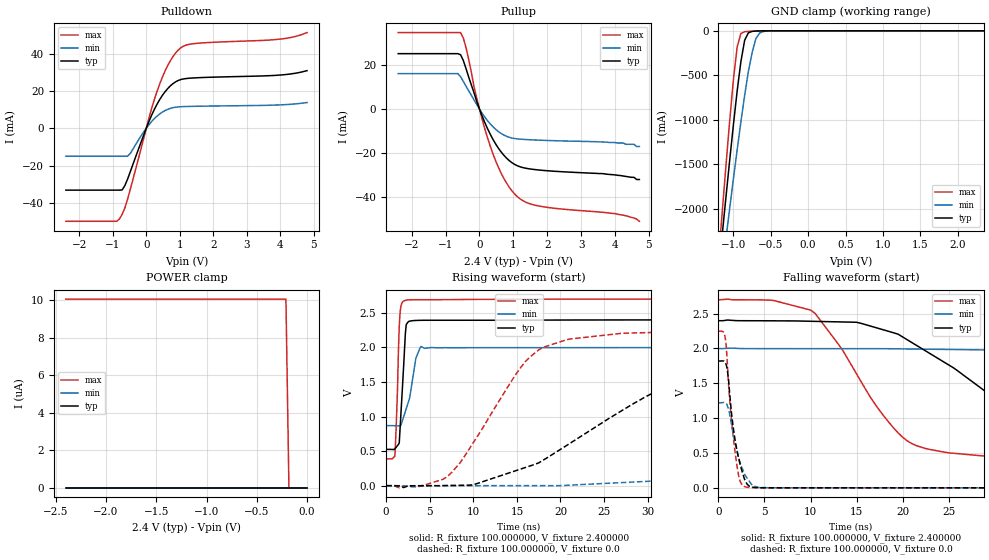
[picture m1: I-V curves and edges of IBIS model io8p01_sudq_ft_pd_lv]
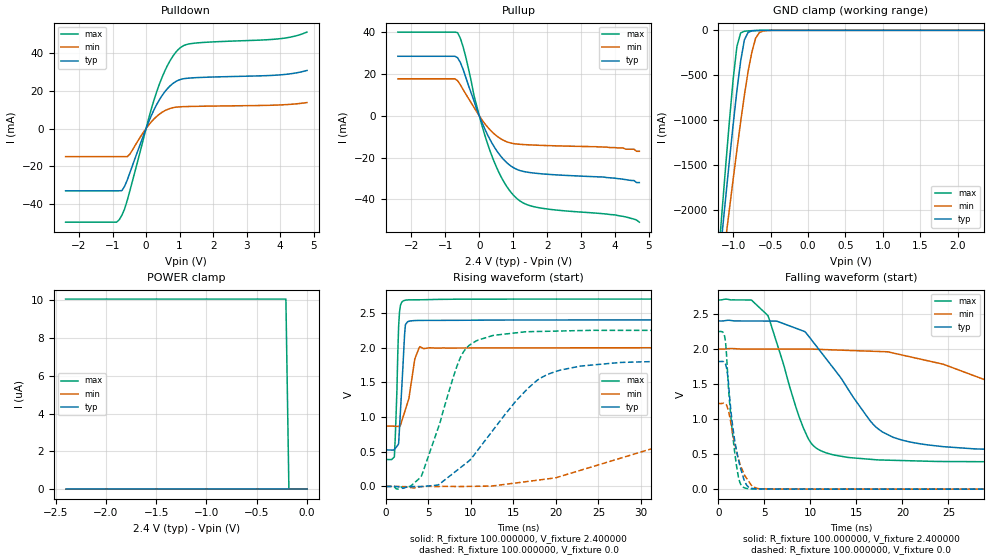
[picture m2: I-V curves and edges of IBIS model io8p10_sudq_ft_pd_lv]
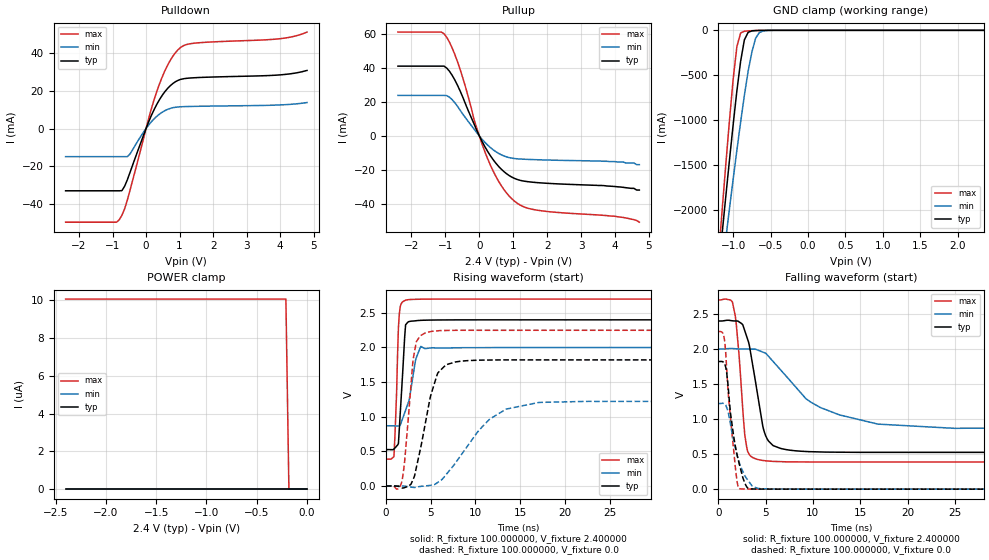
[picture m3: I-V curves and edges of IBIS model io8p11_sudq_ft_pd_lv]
|   stm32f0_444_lqfp32 IBIS Model
[IBIS ver]   4.2
[File name]  stm32f0_444_lqfp32.ibs
[File Rev]   1.0
[Date]   15-5-2013
[Source] Data Created at STMicroelectronics
[Notes]   File originated from ELDO simulations.
[Disclaimer]  This information is for modeling purpose only and is
   not guaranted. The information is subject to change without
   notice.
[Copyright] Copyright 2015 STMicroelectronics Inc.
[Component] stm32f0_444_lqfp32
[Manufacturer] STMicroelectronics
[Package]
| variable   typ   min   max
R_pkg   0.0   NA   NA
L_pkg   0.0H   NA   NA
C_pkg   0.0F   NA   NA
[Pin] signal_name  model_name   R_pin   L_pin   C_pin
1   VDD   POWER   0.03449   2.11E-09   6E-14
2   PF0   io8p_sudq_ft   0.029020556   1.54333E-09   3.22222E-14
3   PF1   io8p_sudq_ft   0.025738889   1.20333E-09   1.55556E-14
4   NRST   ioreset_tc_v33   0.024645   1.09E-09   1E-14
5   VDDA   POWER   0.024645   1.09E-09   1E-14
6   PA0   io8p_sudq_ft   0.025738889   1.20333E-09   1.55556E-14
7   PA1   io8p_sudq_ft   0.029020556   1.54333E-09   3.22222E-14
8   PA2   io8p_sudq_ft   0.03449   2.11E-09   6E-14
9   PA3   io8p_sudq_ft   0.03449   2.11E-09   6E-14
10   PA4   io8p_sudq_ft   0.029020556   1.54333E-09   3.22222E-14
11   PA5   io8p_sudq_ft   0.025738889   1.20333E-09   1.55556E-14
12   PA6   io8p_sudq_ft   0.024645   1.09E-09   1E-14
13   PA7   io8p_sudq_ft   0.024645   1.09E-09   1E-14
14   PB0   io8p_sudq_ft   0.025738889   1.20333E-09   1.55556E-14
15   PB1   io8p_sudq_ft   0.029020556   1.54333E-09   3.22222E-14
16   VSS   GND   0.03449   2.11E-09   6E-14
17   VDD   POWER   0.03449   2.11E-09   6E-14
18   PA8   io8p_sudq_ft   0.029020556   1.54333E-09   3.22222E-14
19   PA9   io8p_sudq_ft   0.025738889   1.20333E-09   1.55556E-14
20   PA10   io8p_sudq_ft   0.024645   1.09E-09   1E-14
21   PA11   io8p_sudq_ft   0.024645   1.09E-09   1E-14
22   PA12   io8p_sudq_ft   0.025738889   1.20333E-09   1.55556E-14
23   PA13   io8p_sudq_ft   0.029020556   1.54333E-09   3.22222E-14
24   PA14   io8p_sudq_ft   0.03449   2.11E-09   6E-14
25   PA15   io8p_sudq_ft   0.03449   2.11E-09   6E-14
26   PB3   io8p_sudq_ft   0.029020556   1.54333E-09   3.22222E-14
27   PB4   io8p_sudq_ft   0.025738889   1.20333E-09   1.55556E-14
28   PB5   io8p_sudq_ft   0.024645   1.09E-09   1E-14
29   PB6   io8p_sudq_i2cin_lv_ft   0.024645   1.09E-09   1E-14
30   PB7   io8p_sudq_i2cin_lv_ft   0.025738889   1.20333E-09   1.55556E-14
31   BOOT0   vpp_test_hv   0.029020556   1.54333E-09   3.22222E-14
32   VSS   GND   0.03449   2.11E-09   6E-14
[Model Selector] io8p_sudq_ft
io8p01_sudq_ft_pd_lv  "SPEED01 2P0V, PD=40kOhm"
io8p01_sudq_ft_pu_lv  "SPEED01 2P0V, PU=40kOhm"
io8p01_sudq_ft_lv  "SPEED01 2P0V"
io8p10_sudq_ft_pd_lv  "SPEED10 2P0V, PD=40kOhm"
io8p10_sudq_ft_pu_lv  "SPEED10 2P0V, PU=40kOhm"
io8p10_sudq_ft_lv  "SPEED10 2P0V"
io8p11_sudq_ft_pd_lv  "SPEED11 2P0V, PD=40kOhm"
io8p11_sudq_ft_pu_lv  "SPEED11 2P0V, PU=40kOhm"
io8p11_sudq_ft_lv  "SPEED11 2P0V"
io8p01_sudq_ft_pd  "SPEED01, PD=40kOhm"
io8p01_sudq_ft_pu  "SPEED01, PU=40kOhm"
io8p01_sudq_ft  "SPEED01"
io8p10_sudq_ft_pd  "SPEED10, PD=40kOhm"
io8p10_sudq_ft_pu  "SPEED10, PU=40kOhm"
io8p10_sudq_ft  "SPEED10"
io8p11_sudq_ft_pd  "SPEED11, PD=40kOhm"
io8p11_sudq_ft_pu  "SPEED11, PU=40kOhm"
io8p11_sudq_ft  "SPEED11"
[Model Selector] io8p_sudq_i2cin_lv_ft
io8p01_sudq_i2cin_lv_ft_pd_lv  "SPEED01 2P0V, PD=40kOhm"
io8p01_sudq_i2cin_lv_ft_pu_lv  "SPEED01 2P0V, PU=40kOhm"
io8p01_sudq_i2cin_lv_ft_lv  "SPEED01 2P0V"
io8p10_sudq_i2cin_lv_ft_pd_lv  "SPEED10 2P0V, PD=40kOhm"
io8p10_sudq_i2cin_lv_ft_pu_lv  "SPEED10 2P0V, PU=40kOhm"
io8p10_sudq_i2cin_lv_ft_lv  "SPEED10 2P0V"
io8p11_sudq_i2cin_lv_ft_pd_lv  "SPEED11 2P0V, PD=40kOhm"
io8p11_sudq_i2cin_lv_ft_pu_lv  "SPEED11 2P0V, PU=40kOhm"
io8p11_sudq_i2cin_lv_ft_lv  "SPEED11 2P0V"
io8p01_sudq_i2cin_lv_ft_pd  "SPEED01, PD=40kOhm"
io8p01_sudq_i2cin_lv_ft_pu  "SPEED01, PU=40kOhm"
io8p01_sudq_i2cin_lv_ft  "SPEED01"
io8p10_sudq_i2cin_lv_ft_pd  "SPEED10, PD=40kOhm"
io8p10_sudq_i2cin_lv_ft_pu  "SPEED10, PU=40kOhm"
io8p10_sudq_i2cin_lv_ft  "SPEED10"
io8p11_sudq_i2cin_lv_ft_pd  "SPEED11, PD=40kOhm"
io8p11_sudq_i2cin_lv_ft_pu  "SPEED11, PU=40kOhm"
io8p11_sudq_i2cin_lv_ft  "SPEED11"
[Model Selector] ioreset_tc_v33
ioreset_tc_v33_pu_lv  "IORESET 2V + PU=40kOhm"
ioreset_tc_v33_nopu_lv  "IORESET 2V"
ioreset_tc_v33_pu  "IORESET + PU=40kOhm"
ioreset_tc_v33_nopu  "IORESET"
[Model Selector] vpp_test_hv
vpp_test_hv_3p3  "Input Buffer"
vpp_test_hv_2p4  "Input Buffer 2P0V"
| Models and submodels in the file (42): io8p01_sudq_ft_pd_lv (I/O), io8p01_sudq_ft_pu_lv (I/O), io8p01_sudq_ft_lv (I/O), io8p10_sudq_ft_pd_lv (I/O), io8p10_sudq_ft_pu_lv (I/O), io8p10_sudq_ft_lv (I/O), io8p11_sudq_ft_pd_lv (I/O), io8p11_sudq_ft_pu_lv (I/O), io8p11_sudq_ft_lv (I/O), io8p01_sudq_ft_pd (I/O), io8p01_sudq_ft_pu (I/O), io8p01_sudq_ft (I/O), io8p10_sudq_ft_pd (I/O), io8p10_sudq_ft_pu (I/O), io8p10_sudq_ft (I/O), io8p11_sudq_ft_pd (I/O), io8p11_sudq_ft_pu (I/O), io8p11_sudq_ft (I/O), io8p01_sudq_i2cin_lv_ft_pd_lv (I/O), io8p01_sudq_i2cin_lv_ft_pu_lv (I/O), io8p01_sudq_i2cin_lv_ft_lv (I/O), io8p10_sudq_i2cin_lv_ft_pd_lv (I/O), io8p10_sudq_i2cin_lv_ft_pu_lv (I/O), io8p10_sudq_i2cin_lv_ft_lv (I/O), io8p11_sudq_i2cin_lv_ft_pd_lv (I/O), io8p11_sudq_i2cin_lv_ft_pu_lv (I/O), io8p11_sudq_i2cin_lv_ft_lv (I/O), io8p01_sudq_i2cin_lv_ft_pd (I/O), io8p01_sudq_i2cin_lv_ft_pu (I/O), io8p01_sudq_i2cin_lv_ft (I/O), io8p10_sudq_i2cin_lv_ft_pd (I/O), io8p10_sudq_i2cin_lv_ft_pu (I/O), io8p10_sudq_i2cin_lv_ft (I/O), io8p11_sudq_i2cin_lv_ft_pd (I/O), io8p11_sudq_i2cin_lv_ft_pu (I/O), io8p11_sudq_i2cin_lv_ft (I/O), ioreset_tc_v33_pu_lv (I/O_open_drain), ioreset_tc_v33_nopu_lv (I/O_open_drain), ioreset_tc_v33_pu (I/O_open_drain), ioreset_tc_v33_nopu (I/O_open_drain), vpp_test_hv_2p4 (Input), vpp_test_hv_3p3 (Input)
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|   Model io8p01_sudq_ft_pd_lv
[Model]  io8p01_sudq_ft_pd_lv
Model_type I/O
Polarity   Non-Inverting
Enable   Active-Low
Vinl =   0.720000V
Vinh =   1.680000V
Vmeas =  1.200000V
Cref =   50.000000pF
Rref =   100.000000M
Vref =   0.0V
C_comp   1.970100pF   1.887900pF   2.069400pF
[Temperature Range]   25.000000   0.125000k   -40.000000
[Pullup Reference]   2.400000V   2.000000V   2.700000V
[Pulldown Reference]   0.0V   0.0V   0.0V
[POWER Clamp Reference]   2.400000V   2.000000V   2.700000V
[GND Clamp Reference]   0.0V   0.0V   0.0V
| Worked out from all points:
|   slope of the pulldown table from 0 to 0.36 V, typ, clamps not added: 25.5 ohm
|   slope of the pullup table from 0 to 0.36 V, typ, clamps not added: 28.4 ohm
|   GND clamp passes 1 mA (typ) near -0.64 V on its own axis
|   rising waveform, R_fixture 100.000000, V_fixture 2.400000: 20-80 % time 499ps typ, 1.06ns min, 336ps max; typ from 0.525 V to 2.4 V
|   rising waveform, R_fixture 100.000000, V_fixture 0.0: 20-80 % time 14.6ns typ, 43.7ns min, 6.88ns max; typ from 0 V to 1.82 V
|   falling waveform, R_fixture 100.000000, V_fixture 2.400000: 20-80 % time 12.9ns typ, 32.5ns min, 7.07ns max; typ from 2.4 V to 0.525 V
|   falling waveform, R_fixture 100.000000, V_fixture 0.0: 20-80 % time 1.15ns typ, 1.36ns min, 910ps max; typ from 1.82 V to 0 V
[Pulldown]
|Voltage   I(typ)   I(min)   I(max)
-2.4V     -33.16mA   -14.98mA   -49.86mA
-880mV    -33.16mA   -14.98mA   -49.86mA
-800mV    -33.16mA   -14.98mA   -48.55mA
-640mV    -30.75mA   -14.98mA   -42.76mA
-480mV    -23.43mA   -13.57mA   -32.92mA
80mV      3.651mA    1.905mA    5.506mA
400mV     15.37mA    7.665mA    23.73mA
720mV     22.75mA    10.69mA    36.23mA
1.04V     26.18mA    11.57mA    43.27mA
1.52V     27.09mA    11.81mA    45.55mA
4V        28.55mA    12.55mA    47.81mA
4.8V      30.9mA     13.81mA    51.31mA
[Pullup]
|Voltage   I(typ)   I(min)   I(max)
-2.4V     25.2mA     16.13mA    34.79mA
-640mV    25.2mA     16.13mA    34.79mA
-560mV    24.71mA    14.75mA    34.79mA
-400mV    18.51mA    10.48mA    28.09mA
-160mV    7.338mA    4.152mA    10.02mA
80mV      -3.229mA   -1.94mA    -4.736mA
400mV     -13.82mA   -8.081mA   -20.45mA
800mV     -22.31mA   -12.38mA   -33.66mA
1.2V      -26.24mA   -13.65mA   -40.83mA
1.76V     -27.69mA   -14.12mA   -44.07mA
4V        -29.9mA    -15.2mA    -47.5mA
4.72V     -32mA      -17mA      -51mA
[GND_clamp]
|Voltage   I(typ)   I(min)   I(max)
-2.4V     -9.788A    -9.782A    -9.734A
-1.2V     -2.718A    -3.021A    -2.568A
-1.15V    -2.29A     -2.675A    -2.036A
-1.1V     -1.868A    -2.333A    -1.515A
-1.05V    -1.454A    -1.995A    -1.012A
-950mV    -674.5mA   -1.337A    -180.6mA
-900mV    -345.2mA   -1.023A    -29.74mA
-850mV    -106.4mA   -726mA     -10.14mA
-750mV    -6.411mA   -244mA     -4.042mA
-700mV    -2.572mA   -88.62mA   -2.346mA
-600mV    -429.6uA   -7.75mA    -383.5uA
2.35V     59.77uA    46.33uA    66.89uA
[POWER_clamp]
|Voltage   I(typ)   I(min)   I(max)
-2.4V     0A         0A         10.06uA
-210mV    0A         0A         10.06uA
-180mV    0A         0A         0A
0V        0A         0A         0A
[Ramp]
| variable   typ   min   max
dV/dt_r  1.09218/14.55718n   0.73266/43.64565n   1.34874/6.87247n
dV/dt_f  1.12429/12.86053n   0.67801/32.45722n   1.38701/7.06387n
R_load = 100.000000
[Rising Waveform]
R_fixture= 100.000000
V_fixture= 2.400000
V_fixture_min= 2.000000
V_fixture_max= 2.700000
|time   V(typ)   V(min)   V(max)
0s        524.8mV    868.7mV    387.2mV
1.001ns   533mV      867mV      427.7mV
1.301ns   579.7mV    865.4mV    1.395V
1.502ns   618.4mV    864.7mV    2.307V
1.602ns   837.8mV    864.4mV    2.512V
2.102ns   1.961V     1.034V     2.677V
2.302ns   2.331V     1.113V     2.684V
3.403ns   2.39V      1.843V     2.691V
4.004ns   2.392V     2.014V     2.691V
49.85ns   2.399V     1.999V     2.699V
[Rising Waveform]
R_fixture= 100.000000
V_fixture= 0.0
V_fixture_min= 0.0
V_fixture_max= 0.0
|time   V(typ)   V(min)   V(max)
0s        1.768nV    15.89nV    1.355nV
7.007ns   1.867mV    822uV      130.1mV
15.02ns   222.8mV    610.6uV    1.635V
17.52ns   330.7mV    351.7uV    1.966V
27.03ns   1.085V     44.44mV    2.204V
34.53ns   1.55V      90.81mV    2.229V
43.04ns   1.723V     239mV      2.246V
84.08ns   1.82V      945.5mV    2.248V
103.1ns   1.82V      1.111V     2.248V
249.2ns   1.82V      1.221V     2.248V
[Falling Waveform]
R_fixture= 100.000000
V_fixture= 2.400000
V_fixture_min= 2.000000
V_fixture_max= 2.700000
|time   V(typ)   V(min)   V(max)
0s        2.399V     1.999V     2.699V
10.01ns   2.391V     1.998V     2.551V
15.02ns   2.376V     1.997V     1.633V
20.02ns   2.165V     1.994V     725.2mV
29.53ns   1.332V     1.979V     449.6mV
35.04ns   877.6mV    1.964V     425.1mV
42.54ns   673.2mV    1.851V     405.8mV
67.07ns   552.7mV    1.286V     389.2mV
85.59ns   536.1mV    1.035V     387.2mV
249.2ns   524.8mV    868.7mV    387.2mV
[Falling Waveform]
R_fixture= 100.000000
V_fixture= 0.0
V_fixture_min= 0.0
V_fixture_max= 0.0
|time   V(typ)   V(min)   V(max)
0s        1.82V      1.221V     2.248V
700.7ps   1.801V     1.221V     2.178V
800.8ps   1.783V     1.214V     2.095V
1.001ns   1.652V     1.164V     1.701V
1.401ns   1.088V     921.6mV    989mV
1.802ns   687.3mV    646.2mV    513.2mV
2.302ns   364.2mV    381.5mV    115.5mV
2.903ns   104.2mV    178.7mV    14.94mV
4.705ns   1.559mV    3.204mV    789.6uV
49.85ns   1.768nV    15.89nV    1.355nV
|   Model io8p10_sudq_ft_pd_lv
[Model]  io8p10_sudq_ft_pd_lv
Model_type I/O
Polarity   Non-Inverting
Enable   Active-Low
Vinl =   0.720000V
Vinh =   1.680000V
Vmeas =  1.200000V
Cref =   50.000000pF
Rref =   100.000000M
Vref =   0.0V
C_comp   1.970100pF   1.887900pF   2.069400pF
[Temperature Range]   25.000000   0.125000k   -40.000000
[Pullup Reference]   2.400000V   2.000000V   2.700000V
[Pulldown Reference]   0.0V   0.0V   0.0V
[POWER Clamp Reference]   2.400000V   2.000000V   2.700000V
[GND Clamp Reference]   0.0V   0.0V   0.0V
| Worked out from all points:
|   slope of the pulldown table from 0 to 0.36 V, typ, clamps not added: 25.5 ohm
|   slope of the pullup table from 0 to 0.36 V, typ, clamps not added: 28.4 ohm
|   GND clamp passes 1 mA (typ) near -0.64 V on its own axis
|   rising waveform, R_fixture 100.000000, V_fixture 2.400000: 20-80 % time 501ps typ, 1.06ns min, 337ps max; typ from 0.525 V to 2.4 V
|   rising waveform, R_fixture 100.000000, V_fixture 0.0: 20-80 % time 7.37ns typ, 21.8ns min, 3.53ns max; typ from 0 V to 1.82 V
|   falling waveform, R_fixture 100.000000, V_fixture 2.400000: 20-80 % time 6.27ns typ, 17.5ns min, 3.34ns max; typ from 2.4 V to 0.525 V
|   falling waveform, R_fixture 100.000000, V_fixture 0.0: 20-80 % time 1.15ns typ, 1.39ns min, 910ps max; typ from 1.82 V to 0 V
[Pulldown]
|Voltage   I(typ)   I(min)   I(max)
-2.4V     -33.16mA   -14.98mA   -49.86mA
-880mV    -33.16mA   -14.98mA   -49.86mA
-800mV    -33.16mA   -14.98mA   -48.55mA
-640mV    -30.75mA   -14.98mA   -42.76mA
-480mV    -23.43mA   -13.57mA   -32.92mA
80mV      3.651mA    1.905mA    5.506mA
400mV     15.37mA    7.665mA    23.73mA
720mV     22.75mA    10.69mA    36.23mA
1.04V     26.18mA    11.57mA    43.27mA
1.52V     27.09mA    11.81mA    45.55mA
4V        28.55mA    12.55mA    47.81mA
4.8V      30.9mA     13.81mA    51.31mA
[Pullup]
|Voltage   I(typ)   I(min)   I(max)
-2.4V     28.56mA    17.75mA    40.16mA
-720mV    28.56mA    17.75mA    40.16mA
-640mV    27.85mA    16.83mA    39.87mA
-480mV    22.39mA    12.66mA    33.22mA
-80mV     3.427mA    2.067mA    4.957mA
160mV     -6.219mA   -3.715mA   -9.137mA
320mV     -11.51mA   -6.781mA   -16.98mA
720mV     -21mA      -11.8mA    -31.53mA
1.12V     -25.77mA   -13.54mA   -39.82mA
1.76V     -27.69mA   -14.12mA   -44.07mA
4V        -29.9mA    -15.2mA    -47.5mA
4.72V     -32mA      -17mA      -51mA
[GND_clamp]
|Voltage   I(typ)   I(min)   I(max)
-2.4V     -9.788A    -9.782A    -9.734A
-1.2V     -2.718A    -3.021A    -2.568A
-1.15V    -2.29A     -2.675A    -2.036A
-1.1V     -1.868A    -2.333A    -1.515A
-1.05V    -1.454A    -1.995A    -1.012A
-950mV    -674.5mA   -1.337A    -180.6mA
-900mV    -345.2mA   -1.023A    -29.74mA
-850mV    -106.4mA   -726mA     -10.14mA
-750mV    -6.411mA   -244mA     -4.042mA
-700mV    -2.572mA   -88.62mA   -2.346mA
-600mV    -429.6uA   -7.75mA    -383.5uA
2.35V     59.77uA    46.33uA    66.89uA
[POWER_clamp]
|Voltage   I(typ)   I(min)   I(max)
-2.4V     0A         0A         10.06uA
-210mV    0A         0A         10.06uA
-180mV    0A         0A         0A
0V        0A         0A         0A
[Ramp]
| variable   typ   min   max
dV/dt_r  1.09206/7.36205n   0.73212/21.76780n   1.34880/3.52140n
dV/dt_f  1.12434/6.26286n   0.67629/17.46251n   1.38699/3.33301n
R_load = 100.000000
[Rising Waveform]
R_fixture= 100.000000
V_fixture= 2.400000
V_fixture_min= 2.000000
V_fixture_max= 2.700000
|time   V(typ)   V(min)   V(max)
0s        524.8mV    868.7mV    387.2mV
1.001ns   532.8mV    867mV      426.6mV
1.301ns   578.6mV    865.5mV    1.387V
1.502ns   616.5mV    864.9mV    2.303V
1.702ns   1.053V     875.4mV    2.602V
2.102ns   1.953V     1.031V     2.676V
2.302ns   2.331V     1.108V     2.683V
3.403ns   2.389V     1.835V     2.689V
4.004ns   2.392V     2.014V     2.689V
49.85ns   2.399V     1.999V     2.699V
[Rising Waveform]
R_fixture= 100.000000
V_fixture= 0.0
V_fixture_min= 0.0
V_fixture_max= 0.0
|time   V(typ)   V(min)   V(max)
0s        1.768nV    15.89nV    1.355nV
2.803ns   -3.26mV    -14.06mV   -1.551mV
4.204ns   -1.822mV   -2.484mV   153.2mV
6.206ns   24.43mV    -1.172mV   860.8mV
8.809ns   274.4mV    -1.373mV   1.867V
12.61ns   812.3mV    7.914mV    2.175V
17.82ns   1.532V     89.58mV    2.232V
23.02ns   1.735V     237.2mV    2.246V
50.05ns   1.82V      1.08V      2.248V
99.7ns    1.82V      1.221V     2.248V
[Falling Waveform]
R_fixture= 100.000000
V_fixture= 2.400000
V_fixture_min= 2.000000
V_fixture_max= 2.700000
|time   V(typ)   V(min)   V(max)
0s        2.399V     1.999V     2.699V
3.604ns   2.399V     1.998V     2.698V
5.405ns   2.398V     1.998V     2.475V
9.61ns    2.218V     1.997V     767.5mV
12.61ns   1.708V     1.986V     485.9mV
17.62ns   835.2mV    1.963V     416.1mV
24.42ns   606.3mV    1.782V     394.4mV
31.83ns   557.1mV    1.421V     389.7mV
47.25ns   529mV      987.2mV    387.3mV
99.7ns    524.8mV    868.7mV    387.2mV
[Falling Waveform]
R_fixture= 100.000000
V_fixture= 0.0
V_fixture_min= 0.0
V_fixture_max= 0.0
|time   V(typ)   V(min)   V(max)
0s        1.82V      1.221V     2.248V
700.7ps   1.8V       1.221V     2.179V
800.8ps   1.783V     1.214V     2.096V
1.001ns   1.653V     1.163V     1.703V
1.401ns   1.09V      921.9mV    991.5mV
1.802ns   688.2mV    647.3mV    514.6mV
2.302ns   364.8mV    386.2mV    116.7mV
2.903ns   104.8mV    188.7mV    16.24mV
4.705ns   2.13mV     3.846mV    2.055mV
49.85ns   1.768nV    15.89nV    1.355nV
|   Model io8p11_sudq_ft_pd_lv
[Model]  io8p11_sudq_ft_pd_lv
Model_type I/O
Polarity   Non-Inverting
Enable   Active-Low
Vinl =   0.720000V
Vinh =   1.680000V
Vmeas =  1.200000V
Cref =   50.000000pF
Rref =   100.000000M
Vref =   0.0V
C_comp   1.970100pF   1.887900pF   2.069400pF
[Temperature Range]   25.000000   0.125000k   -40.000000
[Pullup Reference]   2.400000V   2.000000V   2.700000V
[Pulldown Reference]   0.0V   0.0V   0.0V
[POWER Clamp Reference]   2.400000V   2.000000V   2.700000V
[GND Clamp Reference]   0.0V   0.0V   0.0V
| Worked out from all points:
|   slope of the pulldown table from 0 to 0.36 V, typ, clamps not added: 25.5 ohm
|   slope of the pullup table from 0 to 0.36 V, typ, clamps not added: 28.4 ohm
|   GND clamp passes 1 mA (typ) near -0.64 V on its own axis
|   rising waveform, R_fixture 100.000000, V_fixture 2.400000: 20-80 % time 509ps typ, 1.05ns min, 339ps max; typ from 0.525 V to 2.4 V
|   rising waveform, R_fixture 100.000000, V_fixture 0.0: 20-80 % time 1.79ns typ, 4.5ns min, 864ps max; typ from 0 V to 1.82 V
|   falling waveform, R_fixture 100.000000, V_fixture 2.400000: 20-80 % time 1.38ns typ, 6ns min, 772ps max; typ from 2.4 V to 0.525 V
|   falling waveform, R_fixture 100.000000, V_fixture 0.0: 20-80 % time 1.16ns typ, 1.4ns min, 850ps max; typ from 1.82 V to 0 V
[Pulldown]
|Voltage   I(typ)   I(min)   I(max)
-2.4V     -33.16mA   -14.98mA   -49.86mA
-880mV    -33.16mA   -14.98mA   -49.86mA
-800mV    -33.16mA   -14.98mA   -48.55mA
-640mV    -30.75mA   -14.98mA   -42.76mA
-480mV    -23.43mA   -13.57mA   -32.92mA
80mV      3.651mA    1.905mA    5.506mA
400mV     15.37mA    7.665mA    23.73mA
720mV     22.75mA    10.69mA    36.23mA
1.04V     26.18mA    11.57mA    43.27mA
1.52V     27.09mA    11.81mA    45.55mA
4V        28.55mA    12.55mA    47.81mA
4.8V      30.9mA     13.81mA    51.31mA
[Pullup]
|Voltage   I(typ)   I(min)   I(max)
-2.4V     41.23mA    23.94mA    61.35mA
-1.12V    41.23mA    23.94mA    61.35mA
-960mV    40.07mA    23.8mA     58.26mA
-800mV    35.79mA    21.42mA    51.95mA
-560mV    26.31mA    15.01mA    38.92mA
-160mV    7.338mA    4.152mA    10.02mA
240mV     -8.977mA   -5.327mA   -13.21mA
640mV     -19.51mA   -11.09mA   -29.16mA
1.04V     -25.15mA   -13.38mA   -38.61mA
1.68V     -27.56mA   -14.07mA   -43.82mA
4V        -29.9mA    -15.2mA    -47.5mA
4.72V     -32mA      -17mA      -51mA
[GND_clamp]
|Voltage   I(typ)   I(min)   I(max)
-2.4V     -9.788A    -9.782A    -9.734A
-1.2V     -2.718A    -3.021A    -2.568A
-1.15V    -2.29A     -2.675A    -2.036A
-1.1V     -1.868A    -2.333A    -1.515A
-1.05V    -1.454A    -1.995A    -1.012A
-950mV    -674.5mA   -1.337A    -180.6mA
-900mV    -345.2mA   -1.023A    -29.74mA
-850mV    -106.4mA   -726mA     -10.14mA
-750mV    -6.411mA   -244mA     -4.042mA
-700mV    -2.572mA   -88.62mA   -2.346mA
-600mV    -429.6uA   -7.75mA    -383.5uA
2.35V     59.77uA    46.33uA    66.89uA
[POWER_clamp]
|Voltage   I(typ)   I(min)   I(max)
-2.4V     0A         0A         10.06uA
-210mV    0A         0A         10.06uA
-180mV    0A         0A         0A
0V        0A         0A         0A
[Ramp]
| variable   typ   min   max
dV/dt_r  1.09218/1.79238n   0.73266/4.49807n   1.34886/0.85997n
dV/dt_f  1.12444/1.38128n   0.67760/5.98085n   1.38699/0.77171n
R_load = 100.000000
[Rising Waveform]
R_fixture= 100.000000
V_fixture= 2.400000
V_fixture_min= 2.000000
V_fixture_max= 2.700000
|time   V(typ)   V(min)   V(max)
0s        524.8mV    868.7mV    387.2mV
900.9ps   532.4mV    867.1mV    423.6mV
1.201ns   575.3mV    865.9mV    1.359V
1.401ns   611.4mV    865.5mV    2.286V
1.602ns   1.042V     875.4mV    2.59V
2.202ns   2.327V     1.094V     2.683V
2.603ns   2.374V     1.24V      2.691V
3.303ns   2.385V     1.812V     2.695V
3.904ns   2.392V     2.015V     2.697V
49.85ns   2.399V     1.999V     2.699V
[Rising Waveform]
R_fixture= 100.000000
V_fixture= 0.0
V_fixture_min= 0.0
V_fixture_max= 0.0
|time   V(typ)   V(min)   V(max)
0s        -34.41uV   -16.09uV   -30.77uV
1.802ns   -29.45mV   -740.5uV   67.35mV
3.103ns   111mV      -21.8mV    1.872V
3.403ns   265.9mV    -17.88mV   2.083V
4.505ns   973.4mV    1.615mV    2.214V
5.706ns   1.601V     43.39mV    2.239V
6.707ns   1.75V      161.3mV    2.245V
10.71ns   1.817V     848.5mV    2.248V
13.51ns   1.82V      1.112V     2.248V
49.85ns   1.82V      1.221V     2.248V
[Falling Waveform]
R_fixture= 100.000000
V_fixture= 2.400000
V_fixture_min= 2.000000
V_fixture_max= 2.700000
|time   V(typ)   V(min)   V(max)
0s        2.399V     1.999V     2.699V
1.502ns   2.401V     2.006V     2.669V
1.902ns   2.399V     2.002V     2.364V
2.903ns   2.22V      1.998V     687.3mV
4.004ns   1.477V     1.993V     430.5mV
5.205ns   707.5mV    1.911V     401.7mV
7.508ns   556.9mV    1.561V     389.5mV
10.81ns   530.5mV    1.163V     387.2mV
16.82ns   524.9mV    928.9mV    387.2mV
49.85ns   524.8mV    868.7mV    387.2mV
[Falling Waveform]
R_fixture= 100.000000
V_fixture= 0.0
V_fixture_min= 0.0
V_fixture_max= 0.0
|time   V(typ)   V(min)   V(max)
0s        1.82V      1.221V     2.248V
700.7ps   1.782V     1.213V     2.099V
1.101ns   1.38V      1.068V     1.302V
1.301ns   1.08V      922.8mV    1.007V
1.802ns   621.8mV    592.1mV    322mV
2.102ns   428.2mV    431.4mV    33.52mV
2.302ns   319.1mV    346.1mV    4.266mV
3.103ns   16.96mV    133.5mV    1.213mV
4.605ns   776.8uV    5.445mV    417.8uV
49.85ns   -34.41uV   -16.09uV   -30.77uV
